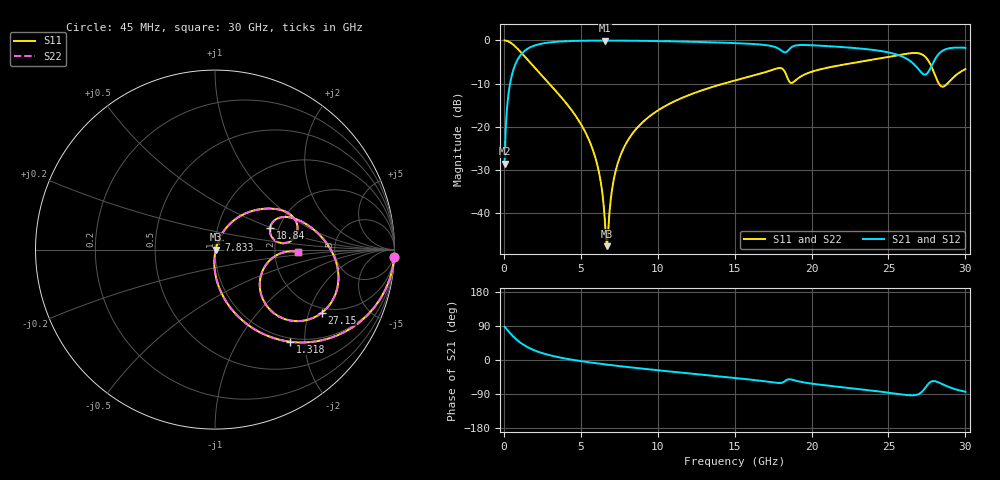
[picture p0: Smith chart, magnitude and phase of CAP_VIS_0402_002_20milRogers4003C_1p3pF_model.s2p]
! S-parameter model data by Modelithics Inc.  support@modelithics.com  813-866-6335  Tampa FL USA
! S-Parameter data specifications:
! Substrate: 20-mil Rogers 4003C, substrate thickness, H=0.508mm, Dielectric constant, Er=3.75
! PCB Mounting Pad Footprint: Pad width, PadW=0.50mm , Pad length, PadL=0.50mm , Pad gap, PadG (edge-to-edge)=0.40mm , Reference planes=1.4mm apart
! Created Wed Nov 18 12:35:58 2015
# hz S ma R 50
! 2 Port Network Data from SP1.SP block
! freq  magS11  angS11  magS21  angS21  magS12  angS12  magS22  angS22
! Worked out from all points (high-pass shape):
!   401 points, 45 MHz to 30 GHz, reference 50 ohm
!   highest |S21| = -0.04 dB at 6.56 GHz (marker M1); lowest = -28.6 dB at 45 MHz (marker M2)
!   |S21| within 3 dB of the highest: 1.169 GHz to 25.3 GHz (24.13 GHz wide, 182 % of centre); 28.3 GHz to end of sweep
!   lowest |S11| = -47.8 dB at 6.71 GHz (marker M3), VSWR 1.01, Z = 50.4 + j0.0112 ohm
!   |S11| at or under -10 dB: 2.935 GHz to 14.31 GHz (11.37 GHz wide, 132 % of centre); 28.27 GHz to 28.84 GHz (564.6 MHz wide, 1.98 % of centre)
!   |S22| runs from -47.8 to 0.0 dB; largest |S21 - S12| = 0
!   S11 on the Smith chart (normalised r, x): 45 MHz: 1, -52; 1.318 GHz: 0.93, -1.70; 7.833 GHz: 1.04, +0.11; 18.84 GHz: 1.80, +0.50; 27.15 GHz: 1.82, -2.45; 30 GHz: 2.73, -0.10
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4.5e7  0.9993 -2.2  0.03717 87.8  0.03717 87.8  0.9993 -2.2
2.696625e8  0.9759 -13.1  0.2179 76.9  0.2179 76.9  0.9759 -13.1
4.94325e8  0.9248 -23.2  0.3799 66.7  0.3799 66.7  0.9248 -23.2
1.318088e9  0.6612 -50.9  0.7488 39.0  0.7488 39.0  0.6612 -50.9
2.666062e9  0.3569 -73.6  0.9317 16.0  0.9317 16.0  0.3569 -73.6
5.062462e9  0.1026 -91.4  0.9912 -3.3  0.9912 -3.3  0.1026 -91.4
6.036e9  0.03801 -93.2  0.9953 -8.8  0.9953 -8.8  0.03801 -93.2
6.33555e9  0.02045 -89.5  0.9958 -10.4  0.9958 -10.4  0.02045 -89.5
6.560212e9  0.008298 -73.3  0.9958 -11.5  0.9958 -11.5  0.008298 -73.3
6.709988e9  0.004093 1.6  0.9958 -12.3  0.9958 -12.3  0.004093 1.6
7.159312e9  0.02521 66.1  0.9954 -14.5  0.9954 -14.5  0.02521 66.1
7.8333e9  0.05856 68.1  0.9937 -17.6  0.9937 -17.6  0.05856 68.1
1.007992e10  0.1568 60.8  0.9823 -27.4  0.9823 -27.4  0.1568 60.8
1.50225e10  0.3429 41.2  0.9309 -47.5  0.9309 -47.5  0.3429 41.2
1.8018e10  0.4767 15.1  0.7678 -60.5  0.7678 -60.5  0.4767 15.1
1.884176e10  0.3306 21.8  0.8611 -53.1  0.8611 -53.1  0.3306 21.8
2.003996e10  0.4351 24.7  0.879 -62.5  0.879 -62.5  0.4351 24.7
2.505742e10  0.646 -0.2  0.7223 -86.6  0.7223 -86.6  0.646 -0.2
2.715428e10  0.6914 -30.5  0.4216 -84.6  0.4216 -84.6  0.6914 -30.5
2.767849e10  0.5481 -44.9  0.459 -59.5  0.459 -59.5  0.5481 -44.9
2.82027e10  0.3337 -41.3  0.675 -58.2  0.675 -58.2  0.3337 -41.3
3e10  0.4649 -1.7  0.8221 -83.7  0.8221 -83.7  0.4649 -1.7
